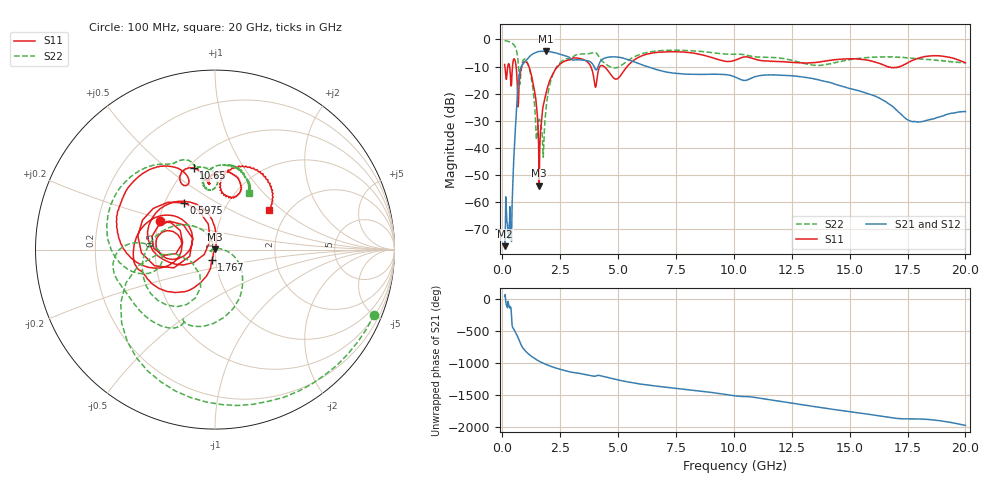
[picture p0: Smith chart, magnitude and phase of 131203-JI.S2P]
!  2-Port S-parameters saved by WinCal
! VAR MeasName=S-Parameters (CALIBRATED_DATA) read from VNA (N5244A)
! VAR MeasDate=4/4/2013 3:53:58 PM
! VAR NAME=131203-JI
! VAR FILENAME=131203-JI.S2P
! VAR DATE=4/4/2013 3:53:58 PM
! VAR PHYS_PORTS=1,2
# Hz S MA R 50
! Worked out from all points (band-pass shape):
!   801 points, 100 MHz to 20 GHz, reference 50 ohm
!   highest |S21| = -4.34 dB at 1.891 GHz (marker M1); lowest = -76.2 dB at 124.9 MHz (marker M2)
!   |S21| within 3 dB of the highest: 1.071 GHz to 2.984 GHz (1.913 GHz wide, 94.4 % of centre); 4.323 GHz to 5.4 GHz (1.078 GHz wide, 22.2 % of centre)
!   lowest |S11| = -53.9 dB at 1.593 GHz (marker M3), VSWR 1.00, Z = 50 + j0.202 ohm
!   |S11| at or under -10 dB: 1.149 GHz to 2.388 GHz (1.239 GHz wide, 70 % of centre); 4.398 GHz to 5.392 GHz (993.7 MHz wide, 20.3 % of centre); 16.61 GHz to 17.15 GHz (542.9 MHz wide, 3.22 % of centre)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
!   |S22| runs from -43.4 to -0.4 dB; largest |S21 - S12| = 0.003
!   S11 on the Smith chart (normalised r, x): 100 MHz: 0.51, +0.18; 597.5 MHz: 0.63, +0.36; 1.767 GHz: 0.96, -0.11; 10.65 GHz: 0.53, +0.62; 20 GHz: 1.60, +0.81
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1e8  0.3457 152.9  0.0002219 43.6  0.0001919 -12.9  0.9569 -22.2
1.24875e8  0.2875 148.5  0.0001556 69.8  0.0009452 16.4  0.9536 -27.4
3.4875e8  0.223 142.0  0.0003368 -120.2  0.000206 -159.5  0.8878 -76.2
5.975e8  0.3123 123.3  0.03932 -176.6  0.03938 -176.1  0.6619 -141.8
7.965e8  0.2677 -165.1  0.2992 15.0  0.2998 15.1  0.226 -110.7
1.14475e9  0.3204 122.7  0.4672 -140.7  0.4684 -140.6  0.3144 161.3
1.44325e9  0.08221 85.0  0.5756 141.1  0.5771 141.0  0.02767 113.1
1.5925e9  0.002021 93.2  0.5995 109.4  0.6012 109.3  0.03378 -153.7
1.766625e9  0.06004 -107.2  0.605 78.2  0.6064 78.2  0.006757 102.1
1.891e9  0.1036 -103.5  0.6067 58.8  0.6083 58.7  0.05409 -3.1
2.33875e9  0.2974 -127.6  0.5596 -0.2  0.5612 -0.3  0.3062 -64.2
3.43325e9  0.436 167.9  0.418 -88.7  0.4192 -88.7  0.5383 -139.1
4.005375e9  0.1396 153.0  0.2896 -125.6  0.2904 -125.7  0.5769 -169.4
4.303875e9  0.3309 171.1  0.423 -124.2  0.4248 -124.5  0.4051 174.9
4.92575e9  0.1858 177.2  0.475 -177.4  0.4765 -177.6  0.3003 -168.8
6.741625e9  0.5803 159.6  0.2723 76.4  0.273 76.0  0.6163 168.0
1.005e10  0.4142 116.8  0.2032 -71.4  0.2033 -71.6  0.5346 114.0
1.0647e10  0.4701 104.7  0.1843 -85.3  0.1842 -85.5  0.5031 105.0
1.338325e10  0.3719 95.8  0.1902 126.2  0.1902 125.8  0.3358 91.2
1.669162e10  0.31 70.3  0.06489 -47.3  0.06546 -47.5  0.4719 78.9
1.783588e10  0.4316 82.1  0.03048 -70.9  0.03038 -71.3  0.4448 68.6
2e10  0.3713 36.0  0.04697 -173.8  0.04724 -173.9  0.3712 59.0
